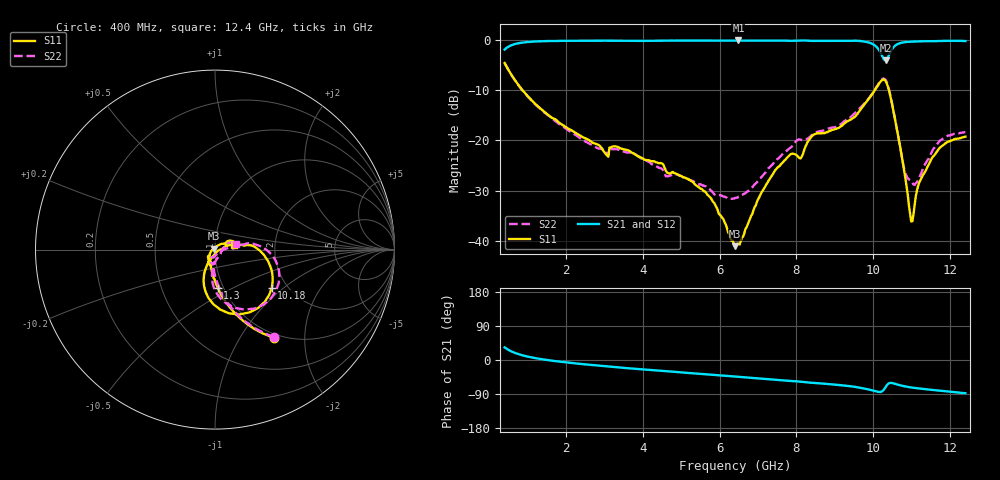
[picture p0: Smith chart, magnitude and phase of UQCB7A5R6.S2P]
!  Part Number  UQCB7A5R6	Mounting Orientation: Vertical
!  Description: RF capacitors
!  Application: Coupling, Bypass, Tuning, DC Block
!  Filters, Matching
# GHZ S DB R 50
! Freq  |S11|  S11 Ph  |S21|  S21 Ph  |S12|  S12 Ph  |S22|  S22 Ph
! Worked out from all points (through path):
!   401 points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, 400 MHz to 12.4 GHz, reference 50 ohm
!   highest |S21| = -0.10 dB at 6.49 GHz (marker M1); lowest = -4.0 dB at 10.33 GHz (marker M2)
!   group delay of S21, straight-line fit = 22.9 ps
!   lowest |S11| = -41.0 dB at 6.4 GHz (marker M3), VSWR 1.02, Z = 49.3 + j0.502 ohm
!   |S11| at or under -10 dB: 866.7 MHz to 10.04 GHz (9.176 GHz wide, 168 % of centre); 10.41 GHz to end of sweep
!   |S22| runs from -31.6 to -4.6 dB; largest |S21 - S12| = 0.0094
!   S11 on the Smith chart (normalised r, x): 400 MHz: 0.94, -1.42; 1.3 GHz: 0.94, -0.42; 10.18 GHz: 1.67, -0.83; 12.4 GHz: 1.23, +0.07
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0.4  -4.59 -56.2  -1.92 33.3  -1.96 33.4  -4.62 -55.9
0.76  -8.97 -73.7  -0.65 15.5  -0.69 15.6  -9.01 -73.0
1.3  -13.41 -85.9  -0.27 3.2  -0.32 3.3  -13.53 -84.1
2.41  -19.24 -100.7  -0.15 -10.7  -0.19 -10.6  -19.80 -93.5
3.04  -22.77 -111.3  -0.15 -16.5  -0.18 -16.3  -22.33 -95.1
3.31  -21.20 -108.1  -0.15 -19.0  -0.18 -18.8  -21.74 -99.7
4.42  -24.53 -127.3  -0.15 -28.0  -0.18 -27.7  -25.45 -111.3
5.68  -30.82 -149.4  -0.14 -38.0  -0.15 -37.6  -29.44 -88.4
6.4  -41.03 145.0  -0.10 -43.6  -0.11 -43.3  -31.44 -44.6
6.49  -40.56 118.8  -0.10 -44.4  -0.10 -44.0  -31.19 -37.6
7.42  -26.25 41.2  -0.12 -51.9  -0.10 -51.5  -24.30 4.7
8.11  -23.56 26.6  -0.11 -57.3  -0.09 -56.9  -19.85 3.0
8.41  -19.11 24.4  -0.19 -60.1  -0.16 -59.7  -18.89 6.7
9.73  -13.24 4.4  -0.28 -74.6  -0.23 -74.2  -13.00 7.7
10.18  -8.38 -33.9  -2.39 -84.4  -2.35 -84.0  -8.22 -22.5
10.33  -8.27 -69.5  -4.05 -70.2  -4.00 -69.8  -8.06 -56.2
10.42  -10.33 -91.7  -2.83 -61.0  -2.79 -60.7  -10.14 -77.4
10.81  -26.24 -112.0  -0.45 -69.3  -0.44 -69.1  -25.74 -76.5
10.99  -36.12 -57.5  -0.34 -72.5  -0.33 -72.3  -28.23 -36.9
11.2  -28.37 4.2  -0.27 -75.2  -0.25 -75.1  -27.41 6.0
11.56  -23.20 18.2  -0.25 -79.1  -0.23 -79.0  -21.72 26.3
12.4  -19.24 14.1  -0.22 -87.8  -0.20 -87.7  -18.33 15.7
